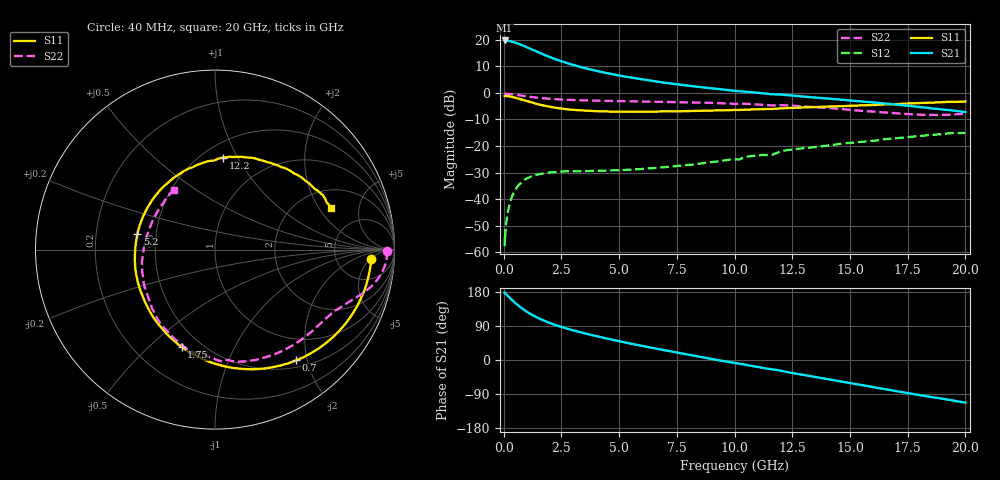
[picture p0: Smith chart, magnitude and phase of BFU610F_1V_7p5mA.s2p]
! Filename:  P:\Prog\Test\Noise\ATS_data\Testdata_Net\SplitFiles\BFU610_2W_A5_HighFreq_1V_7.5mA_D.s2p
! Date/Time: Wed 10/Aug/2011 16:54:54
! BFU610_2W_A5_HighFreq_1V_1mA_10mA_Bias5_R.s2p
! MDIF S-parameter v. bias file
! BFU610_2W_A5_HighFreq_1V_1mA_10mA
! Date/time Mon Aug 08 13:53:02 2011
! VAR V_out= 1.0000
! VAR I_out= 7.4950
! VAR V_in= 0.9313
! VAR I_in= 0.0700
! Device data file deembeded for feedlines and parallel
! Original file: \SplitFiles\BFU610_2W_A5_HighFreq_1V_7.5mA_R.s2p
! Feed-files: PR003V01_101208_Feed1.s2p, PR003V01_101208_Feed2.s2p
! Parallel-file: PR003V01_101208_Par.s2p
# MHz S MA R 50
!  Freq-MHz  S11-mag  S11-arg  S21-mag  S21-arg  S12-mag  S12-arg  S22-mag  S22-arg
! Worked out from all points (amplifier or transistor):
!   167 points, 40 MHz to 20 GHz, reference 50 ohm
!   highest |S21| = 19.7 dB at 40 MHz (marker M1)
!   |S21| within 3 dB of that: start of sweep to 1.114 GHz
!   unconditionally stable (mu >= 1): 1.975 GHz to end of sweep
!   at 550 MHz: K = 0.32, MSG = 27.3 dB, |S12| = -35.9 dB
!   at 4.2 GHz: K = 2.24, MAG = 12.3 dB, |S12| = -29.3 dB
!   at 20 GHz: K = 2.84, MAG = -3.5 dB, |S12| = -15.1 dB
!   S11 on the Smith chart (normalised r, x): 40 MHz: 12, -5; 700 MHz: 0.61, -1.81; 1.75 GHz: 0.40, -0.64; 5.2 GHz: 0.39, +0.09; 12.2 GHz: 0.62, +0.87; 20 GHz: 2.94, +2.60
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40  0.8725 -3.3  9.664 177.7  0.001301 76.9  0.9588 -0.5
50  0.8721 -4.1  9.634 177.3  0.002137 75.1  0.9596 -0.8
160  0.8652 -13.1  9.54 170.2  0.005079 79.9  0.9573 -3.3
260  0.8534 -21.2  9.41 164.2  0.008196 76.5  0.9507 -5.4
400  0.8295 -32.2  9.089 156.1  0.01225 70.7  0.9368 -8.1
550  0.7993 -43.4  8.668 147.9  0.01609 64.3  0.9176 -10.7
700  0.7651 -53.8  8.182 140.6  0.01942 58.6  0.8971 -13.0
950  0.709 -69.7  7.359 129.5  0.02377 50.6  0.8636 -16.1
1250  0.6491 -86.2  6.438 118.4  0.02726 43.1  0.8289 -18.9
1500  0.6068 -98.3  5.77 110.5  0.02933 38.1  0.8057 -20.9
1750  0.573 -108.9  5.196 103.7  0.0307 34.2  0.7867 -22.7
2050  0.5395 -120.2  4.61 96.4  0.03184 30.6  0.7694 -24.8
2500  0.5045 -134.8  3.921 87.1  0.03295 26.9  0.7467 -27.6
3400  0.4659 -157.7  3.004 72.0  0.03345 23.3  0.7227 -33.3
4200  0.4487 -174.2  2.483 60.2  0.03429 22.8  0.7083 -38.6
5200  0.4414 168.4  2.036 47.1  0.03531 24.5  0.6954 -45.7
6800  0.4437 145.1  1.585 27.7  0.03923 28.6  0.6758 -57.5
10200  0.4756 104.7  1.067 -9.6  0.05543 34.2  0.6193 -83.9
12200  0.5147 85.1  0.9122 -30.7  0.08233 30.6  0.5819 -103.2
13400  0.5386 73.8  0.8189 -43.7  0.09424 22.3  0.5381 -116.6
16800  0.6099 45.0  0.6137 -80.0  0.137 0.3  0.4184 -166.3
20000  0.6875 19.9  0.4343 -112.5  0.1764 -29.7  0.4046 124.2
